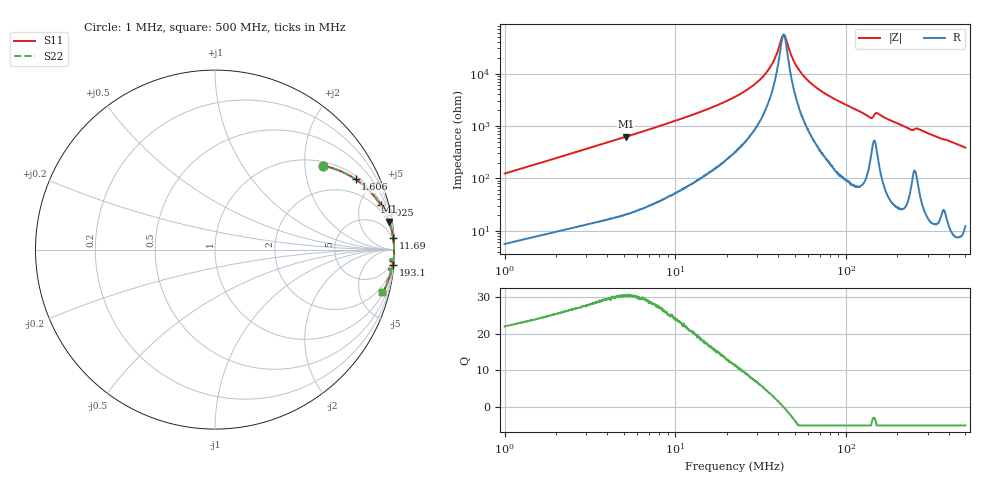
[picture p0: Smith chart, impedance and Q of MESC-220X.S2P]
!s-Parameter Generated by FASTRON Sdn. Bhd.
!FASTRON P/N : MESC-220X
!Keysight Technologies,E4991B,MY54100416,A.01.15
!Date: Mon Mar 16 11:11:46 2026
!Version  : Rev00 Mon Mar 16 11:11:46 2026
!Data & Calibration Information:
!PortZ  Port1:50+j0  Port2:50+j0
!When reading, reference impedance value at option line is always used.
! Remarks : This data is being provided solely for informational purposes.
!Freq	S11	S21	S12	S22
# Hz S dB R 50
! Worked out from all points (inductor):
!   1601 points, 1 MHz to 500 MHz, reference 50 ohm
!   read as one part in series: L = 19.5 uH near 1.032 MHz
!   highest Q = 30.4 at 5.151 MHz (marker M1), where L = 19.2 uH
!   self-resonance near 42.94 MHz
!   S11 on the Smith chart (normalised r, x): 1 MHz: 1.11, +2.46; 1.606 MHz: 1.16, +3.91; 3.025 MHz: 1.26, +7.29; 11.69 MHz: 2, +30; 193.1 MHz: 2, -23; 500 MHz: 1.24, -7.72
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1000000  -2.38 38.0  -4.21 -49.4  -4.21 -49.4  -2.38 38.0
1606188  -1.15 26.6  -6.98 -61.1  -6.98 -61.1  -1.15 26.6
2820919  -0.45 16.2  -11.08 -71.7  -11.08 -71.7  -0.45 16.2
3025200  -0.39 15.2  -11.63 -72.7  -11.63 -72.7  -0.39 15.2
5150547  -0.16 9.1  -16.04 -79.0  -16.04 -79.0  -0.16 9.1
7957584  -0.08 5.8  -19.90 -82.1  -19.90 -82.1  -0.08 5.8
1.168907e7  -0.05 3.8  -23.54 -83.5  -23.54 -83.5  -0.05 3.8
2.236068e7  -0.02 1.6  -31.10 -83.4  -31.10 -83.4  -0.02 1.6
2.855992e7  -0.02 1.0  -35.44 -81.6  -35.44 -81.6  -0.02 1.0
3.401461e7  -0.02 0.5  -40.22 -77.3  -40.22 -77.3  -0.02 0.5
3.762909e7  -0.02 0.3  -44.76 -69.9  -44.76 -69.9  -0.02 0.3
4.195229e7  -0.02 0.1  -53.53 -29.6  -53.53 -29.6  -0.02 0.1
4.310858e7  -0.02 -0.0  -54.76 1.5  -54.76 1.5  -0.02 -0.0
4.429673e7  -0.02 -0.1  -53.60 31.8  -53.60 31.8  -0.02 -0.1
4.7875e7  -0.02 -0.2  -46.75 67.5  -46.75 67.5  -0.02 -0.2
5.134194e7  -0.01 -0.4  -42.77 76.8  -42.77 76.8  -0.01 -0.4
6.307767e7  -0.01 -0.9  -35.99 83.6  -35.99 83.6  -0.01 -0.9
1.371661e8  -0.09 -3.8  -23.40 79.1  -23.40 79.1  -0.09 -3.8
1.517418e8  -0.10 -3.2  -24.98 76.5  -24.98 76.5  -0.10 -3.2
1.77937e8  -0.05 -4.3  -22.46 83.9  -22.46 83.9  -0.05 -4.3
1.930591e8  -0.05 -4.9  -21.45 83.7  -21.45 83.7  -0.05 -4.9
5e8  -0.35 -14.4  -12.09 73.8  -12.09 73.8  -0.35 -14.4
